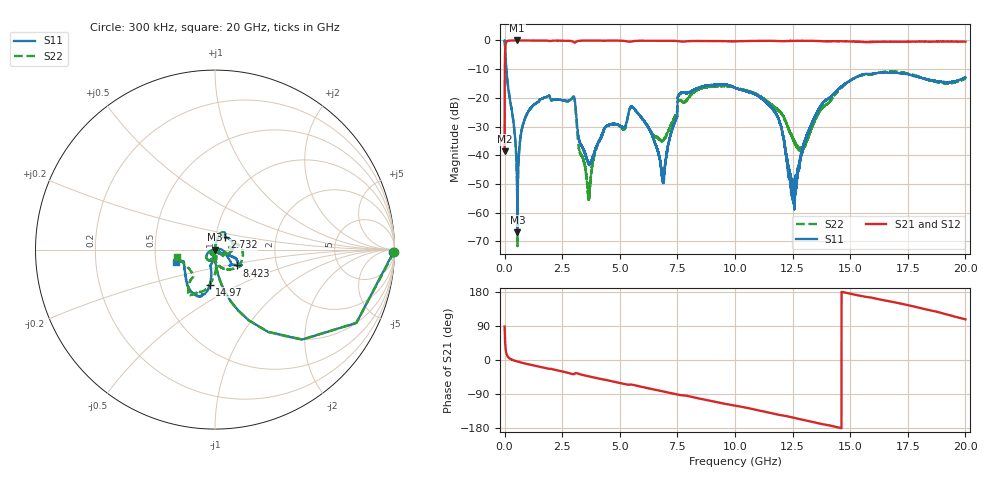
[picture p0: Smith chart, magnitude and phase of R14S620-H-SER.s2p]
!{R14S620}
!Johanson Technology Inc.
!www.johansontechnology.com
!Test Board Conditions:
!Substrate Type  RO4350B
!Substrate Thickness  20 mil
!Substrate Dk  3.66
!TL Type: GCPW
!TL Trace Width  36 mil
!TL Gap  12 mil
!Electrode orientation  Horizontal
!DUT TOPOLOGY	SERIES
!Mounting Pad LxW  26x36 mil
! Created Wed Nov 25 17:33:21 2020
! 2 Port Network Data from SP1.SP block
! freq  magS11  angS11  magS21  angS21  magS12  angS12  magS22  angS22
# khz S ma R 50
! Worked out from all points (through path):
!   20001 points, 300 kHz to 20 GHz, reference 50 ohm
!   highest |S21| = 0.00 dB at 547.3 MHz (marker M1); lowest = -38.6 dB at 300 kHz (marker M2)
!   group delay of S21, straight-line fit = 34.9 ps
!   lowest |S11| = -66.9 dB at 558.3 MHz (marker M3), VSWR 1.00, Z = 50 + j0.0137 ohm
!   |S11| at or under -10 dB: 75.62 MHz to end of sweep
!   |S22| runs from -71.7 to 0.0 dB; largest |S21 - S12| = 0.018
!   S11 on the Smith chart (normalised r, x): 300 kHz: open; 2.732 GHz: 1.10, +0.16; 8.423 GHz: 1.25, -0.23; 14.97 GHz: 0.88, -0.36; 20 GHz: 0.64, -0.09
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300  0.9937 -0.9  0.01169 88.2  0.01162 89.3  0.9978 -0.8
112300  0.2148 -78.3  0.9761 11.6  0.9752 11.5  0.2159 -78.4
547300  0.001952 -84.0  1 -3.9  0.9991 -3.9  0.001868 -102.5
558300  0.0004522 17.6  0.9994 -4.1  0.9991 -4.1  0.0002833 177.1
1121300  0.06543 76.3  0.9964 -12.5  0.9975 -12.6  0.06474 78.2
2732300  0.08821 53.1  0.9893 -33.5  0.9895 -33.5  0.08749 53.4
3006300  0.1054 13.1  0.9269 -37.3  0.9278 -37.3  0.1019 12.0
3334300  0.01476 8.0  0.9905 -38.6  0.9914 -38.5  0.00999 29.4
3658300  0.007178 -31.0  0.9954 -43.2  0.994 -43.2  0.001896 139.2
4356300  0.03027 -116.4  0.99 -52.1  0.9901 -52.1  0.03007 -142.1
5532300  0.06959 -125.4  0.9644 -65.2  0.964 -65.2  0.06921 -131.7
6667300  0.01109 -169.1  0.9891 -80.2  0.9888 -80.2  0.01976 -108.7
6892300  0.00359 90.3  0.9907 -83.0  0.9906 -83.1  0.01829 -76.9
7600300  0.1162 -39.6  0.964 -92.4  0.9643 -92.4  0.08987 6.2
8423300  0.15 -36.2  0.9784 -101.4  0.9772 -101.3  0.1398 8.3
1.00003e7  0.1499 -30.3  0.9642 -120.2  0.9651 -120.2  0.1492 -45.3
1.17943e7  0.05207 -30.0  0.9789 -143.3  0.9803 -143.2  0.0653 -94.2
1.25273e7  0.003807 -40.8  0.9847 -152.0  0.9849 -152.0  0.01917 -141.2
1.33343e7  0.03568 -102.0  0.9831 -163.0  0.9841 -163.0  0.03021 -79.0
1.49713e7  0.1972 -98.5  0.9625 175.4  0.9629 175.1  0.1978 -98.8
1.66673e7  0.2734 -111.9  0.9525 155.3  0.9448 155.0  0.2896 -118.7
2e7  0.2277 -162.4  0.9495 107.2  0.9492 107.3  0.2184 -169.1
